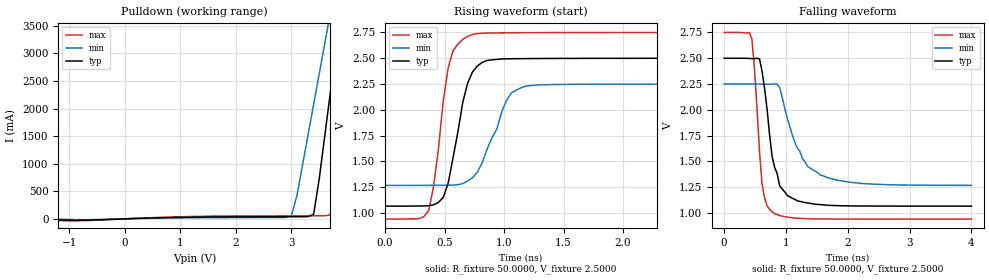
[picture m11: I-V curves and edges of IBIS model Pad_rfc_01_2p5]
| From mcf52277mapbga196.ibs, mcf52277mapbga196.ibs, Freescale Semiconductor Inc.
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|   Model Pad_rfc_01_2p5
[Model]   Pad_rfc_01_2p5
Model_type   Open_drain
Polarity   Non-Inverting
Enable   Active-High
Vmeas =   1.2500V
C_comp   1.7450pF   1.6200pF   1.8900pF
[Temperature Range]   25.0000   0.1500k   -40.0000
[Voltage Range]   2.5000V   2.2500V   2.7500V
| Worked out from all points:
|   slope of the pulldown table from 0 to 0.375 V, typ, clamps not added: 29.5 ohm
|   rising waveform, R_fixture 50.0000, V_fixture 2.5000: 20-80 % time 143ps typ, 200ps min, 115ps max; typ from 1.07 V to 2.5 V
|   falling waveform, R_fixture 50.0000, V_fixture 2.5000: 20-80 % time 215ps typ, 371ps min, 119ps max; typ from 2.5 V to 1.07 V
[Pulldown]
| voltage   I(typ)   I(min)   I(max)
-2.5V     -830uA     -550uA     -1mA
-900mV    -27.33mA   -13.6mA    -36.25mA
3V        38.48mA    59.01mA    54.49mA
3.1V      38.58mA    425.9mA    54.62mA
3.4V      84.25mA    2.073A     54.98mA
3.5V      719.9mA    2.624A     55.1mA
3.6V      1.499A     3.175A     55.33mA
3.7V      2.278A     3.726A     72.43mA
3.8V      3.059A     4.278A     758.3mA
4V        4.622A     5.383A     2.751A
4.2V      6.188A     6.489A     4.747A
5V        12.47A     10.92A     12.76A
[Ramp]
| variable   typ   min   max
dV/dt_r   0.8603/0.1372n   0.5896/0.1946n   1.0856/0.1123n
dV/dt_f   0.8603/0.2085n   0.5896/0.3830n   1.0856/0.1259n
R_load = 50.0000
[Rising Waveform]
R_fixture = 50.0000
V_fixture = 2.5000
V_fixture_min = 2.2500
V_fixture_max = 2.7500
| time   V(typ)   V(min)   V(max)
0s        1.066V     1.267V     940.7mV
367.3ps   1.07V      1.267V     1.024V
408.2ps   1.078V     1.268V     1.258V
530.6ps   1.289V     1.268V     2.409V
571.4ps   1.536V     1.27V      2.574V
693.9ps   2.258V     1.31V      2.712V
816.3ps   2.46V      1.485V     2.741V
1.02ns    2.494V     2.09V      2.747V
1.184ns   2.497V     2.23V      2.748V
4ns       2.5V       2.25V      2.75V
[Falling Waveform]
R_fixture = 50.0000
V_fixture = 2.5000
V_fixture_min = 2.2500
V_fixture_max = 2.7500
| time   V(typ)   V(min)   V(max)
0s        2.5V       2.25V      2.75V
449ps     2.496V     2.25V      2.686V
612.2ps   2.38V      2.248V     1.285V
693.9ps   2.009V     2.248V     1.069V
816.3ps   1.443V     2.25V      992.3mV
898ps     1.263V     2.215V     974.4mV
1.02ns    1.169V     1.921V     960.4mV
1.265ns   1.106V     1.528V     945.9mV
1.551ns   1.081V     1.37V      941.8mV
4ns       1.066V     1.267V     940.7mV
